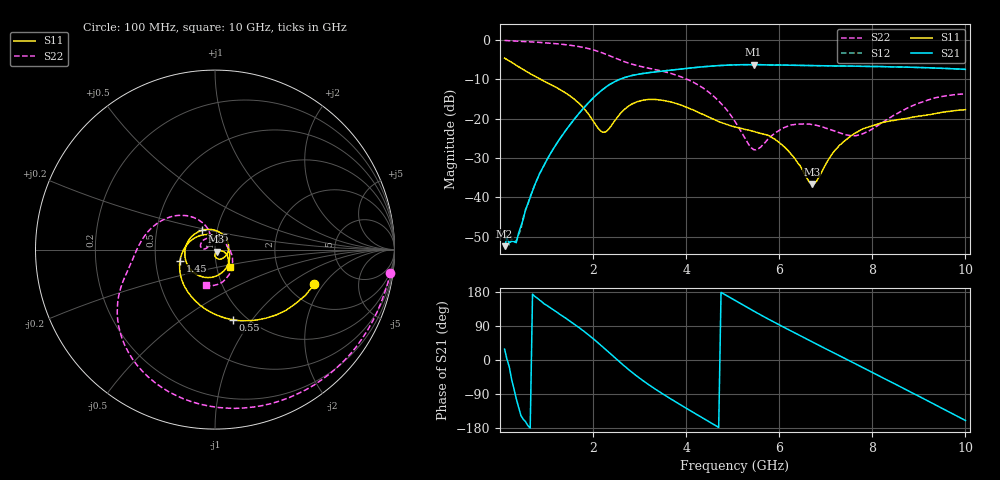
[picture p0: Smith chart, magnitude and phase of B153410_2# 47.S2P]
!  2-Port S-parameters saved by WinCal
! VAR MeasName=S-Parameters (CALIBRATED_DATA) read from VNA (N5245A)
! VAR MeasDate=2016-12-23 10:01:47
! VAR NAME=B153410_2# 47
! VAR FILENAME=B153410_2# 47.S2P
! VAR DATE=2016-12-23 10:01:47
! VAR PHYS_PORTS=1,2
# Hz S DB R 50
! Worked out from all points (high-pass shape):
!   199 points, 100 MHz to 10 GHz, reference 50 ohm
!   highest |S21| = -6.28 dB at 5.45 GHz (marker M1); lowest = -52.4 dB at 100 MHz (marker M2)
!   |S21| within 3 dB of the highest: 2.757 GHz to end of sweep
!   lowest |S11| = -36.6 dB at 6.7 GHz (marker M3), VSWR 1.03, Z = 50.8 - j1.23 ohm
!   |S11| at or under -10 dB: 871 MHz to end of sweep
!   |S22| runs from -27.9 to -0.1 dB; largest |S21 - S12| = 0.0027
!   S11 on the Smith chart (normalised r, x): 100 MHz: 2.78, -1.64; 550 MHz: 0.87, -0.81; 1.45 GHz: 0.67, -0.09; 4.15 GHz: 0.85, +0.19; 10 GHz: 1.16, -0.23
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1e8  -4.63 -19.2  -52.39 28.7  -50.68 33.4  -0.13 -7.5
1.5e8  -4.97 -26.8  -50.32 2.1  -49.73 -6.7  -0.17 -10.9
2e8  -5.34 -33.7  -51.49 -17.9  -52.02 -16.8  -0.22 -14.3
3.5e8  -6.45 -53.3  -51.50 -102.1  -51.05 -109.9  -0.31 -24.3
5.5e8  -7.88 -75.6  -43.09 -162.9  -43.26 -167.4  -0.42 -37.5
1e9  -10.79 -118.6  -30.65 144.6  -30.62 145.0  -0.75 -66.8
1.45e9  -13.77 -162.2  -22.40 107.2  -22.41 107.2  -1.26 -95.5
1.75e9  -16.68 161.5  -17.94 80.9  -17.94 81.0  -1.81 -114.5
2.25e9  -23.45 37.1  -12.20 30.1  -12.21 30.2  -3.52 -144.4
2.75e9  -16.92 -81.8  -9.30 -23.8  -9.28 -23.6  -5.83 -165.0
3.4e9  -15.20 -159.7  -8.05 -81.8  -8.01 -81.8  -7.70 173.0
4.15e9  -17.79 123.3  -7.06 -138.1  -7.06 -138.1  -10.72 139.7
4.6e9  -20.20 70.0  -6.59 -170.7  -6.60 -170.7  -14.39 119.2
5.05e9  -22.10 12.3  -6.33 157.0  -6.34 157.2  -20.72 107.8
5.45e9  -23.22 -32.5  -6.28 129.3  -6.28 129.4  -27.86 139.7
6.1e9  -27.06 -83.3  -6.40 86.4  -6.39 86.4  -22.30 172.2
6.7e9  -36.60 -55.0  -6.51 48.4  -6.53 48.4  -21.48 144.0
7.4e9  -25.70 -13.8  -6.64 4.8  -6.63 4.8  -23.96 84.9
7.75e9  -22.88 -23.4  -6.71 -17.2  -6.69 -17.0  -24.06 40.4
8.35e9  -20.66 -37.1  -6.83 -54.8  -6.81 -54.5  -19.93 -19.7
9.15e9  -19.13 -44.6  -7.04 -105.2  -7.06 -105.1  -15.43 -66.8
1e10  -17.71 -49.9  -7.48 -159.6  -7.48 -159.3  -13.75 -104.2
